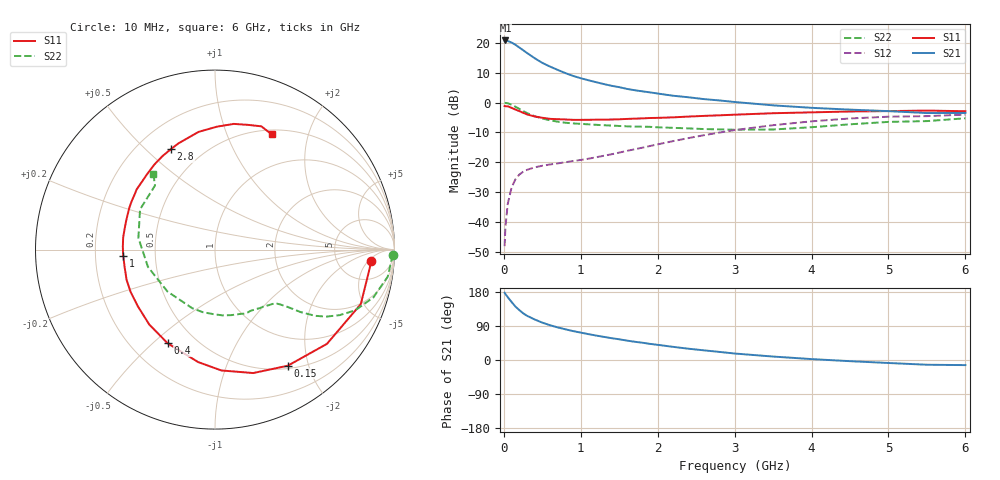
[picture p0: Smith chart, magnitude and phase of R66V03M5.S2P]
! SIEMENS Small Signal Semiconductors
! BFR193
! Si NPN RF Bipolar Junction Transistor in SOT23
! VCE = 6 V  IC = 3.5 mA
! Common Emitter S-Parameters:  May  1996
# GHz  S  MA  R  50
!  f  S11  S21  S12  S22
! GHz  MAG  ANG  MAG  ANG  MAG  ANG  MAG  ANG
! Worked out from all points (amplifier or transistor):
!   36 points, 10 MHz to 6 GHz, reference 50 ohm
!   highest |S21| = 20.8 dB at 20 MHz (marker M1)
!   |S21| within 3 dB of that: start of sweep to 236.2 MHz
!   unconditionally stable (mu >= 1): 1.015 GHz to 2.03 GHz
!   at 250 MHz: K = 0.33, MSG = 20.4 dB, |S12| = -23.2 dB
!   at 1.4 GHz: K = 1.08, MAG = 9.7 dB, |S12| = -17.3 dB
!   at 6 GHz: K = 0.97, MSG = 0.3 dB, |S12| = -4.0 dB
!   S11 on the Smith chart (normalised r, x): 10 MHz: 12, -6; 150 MHz: 0.54, -1.68; 400 MHz: 0.35, -0.56; 1 GHz: 0.32, -0.03; 2.8 GHz: 0.34, +0.60; 6 GHz: 0.55, +1.46
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0.01  0.8733 -4.1  10.96 177.4  0.0039 87.6  0.9941 -1.7
0.02  0.8657 -8.4  11.01 174.2  0.0079 85.5  0.9842 -3.7
0.05  0.8672 -20.5  10.79 166.1  0.0197 78.6  0.9742 -8.9
0.1  0.8154 -40.1  10.17 153.3  0.0374 69.8  0.9216 -16.8
0.15  0.7635 -57.9  9.325 141.1  0.0514 61.0  0.8516 -23.4
0.2  0.72 -72.8  8.41 131.9  0.0618 55.5  0.7852 -27.7
0.25  0.6743 -87.0  7.57 123.4  0.069 50.5  0.7229 -31.1
0.3  0.6337 -98.5  6.809 116.8  0.0743 47.6  0.6682 -33.5
0.4  0.5849 -116.8  5.553 107.0  0.0819 43.6  0.5912 -36.1
0.5  0.5553 -131.3  4.631 98.6  0.0871 42.0  0.5403 -37.5
0.6  0.5334 -143.7  4.017 91.8  0.0915 42.3  0.5042 -38.7
0.7  0.526 -153.4  3.529 86.0  0.0954 43.3  0.478 -39.9
0.8  0.5205 -161.2  3.121 81.0  0.0998 44.3  0.4591 -41.0
1  0.5126 -176.0  2.558 72.2  0.109 48.0  0.4391 -43.8
1.1  0.5138 178.2  2.365 68.3  0.1143 49.8  0.4313 -45.9
1.6  0.5315 153.8  1.695 51.2  0.1546 57.8  0.3992 -57.2
2.2  0.5648 132.3  1.302 34.7  0.2256 59.7  0.3766 -75.7
2.8  0.6109 113.8  1.086 21.4  0.3132 54.8  0.3552 -101.1
3.5  0.6624 97.9  0.898 9.1  0.4172 43.8  0.353 -138.6
4.5  0.7081 81.5  0.761 -3.1  0.541 25.7  0.4318 171.3
5.5  0.7337 69.4  0.667 -12.5  0.592 7.5  0.489 133.1
6  0.7157 63.8  0.67 -13.5  0.6281 2.4  0.5446 129.1
